FUNCTION_BLOCK FB_VibrationSource
VAR_INPUT
	x: LREAL;
END_VAR
VAR_OUTPUT
	vib: LREAL;
END_VAR
VAR
	a : ARRAY[0..9] OF LREAL;
	b : ARRAY[0..9] OF LREAL;
	c : LREAL;
	i: INT;
	sig : LREAL;
END_VAR

sig := 0;
FOR i := 0 TO 9 BY 1 DO
	sig := sig + a[i] * COS(b[i]*x/c *  2 * PI);
END_FOR

vib := sig;

METHOD FB_init : BOOL
VAR_INPUT
	bInitRetains : BOOL; // if TRUE, the retain variables are initialized (warm start / cold start)
	bInCopyCode : BOOL;  // if TRUE, the instance afterwards gets moved into the copy code (online change)
	Amplitude : ARRAY[0..9] OF LREAL;
	Harmonic : ARRAY[0..9] OF LREAL;
	fPositionScaling  : LREAL;
END_VAR
a:= Amplitude;
b:= Harmonic;
c:= fPositionScaling;
END_METHOD

END_FUNCTION_BLOCK
